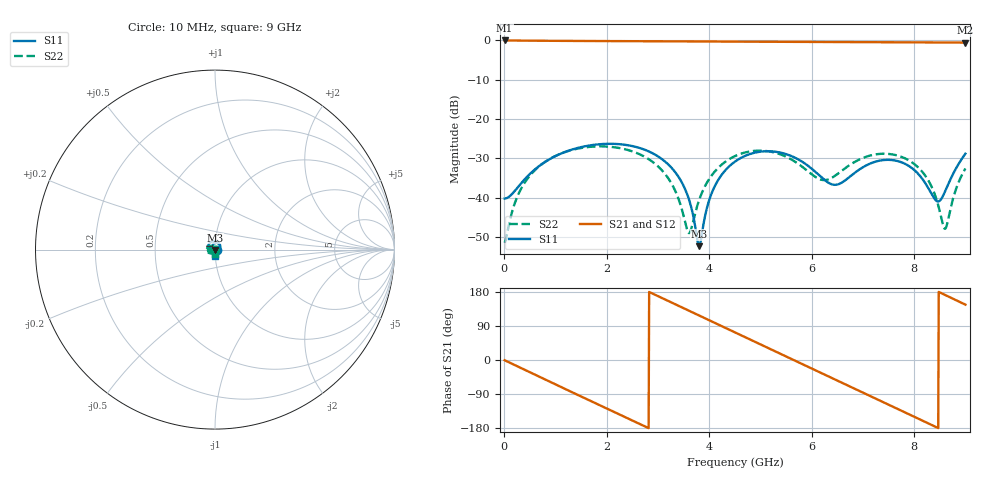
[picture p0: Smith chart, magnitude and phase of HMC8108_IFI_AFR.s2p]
! Analog Devices, Inc.
! 1 Analog Way
! Wilmington, MA 01887
! http://www.analog.com
! Date:  2021-09-07 NN
! Board Name:  EV1HMC8108LC5 Revision A with HMC8108LC5 installed
! File Description:  Automatic Fixture Removal S-Parameters for IFI Port connector and board loss de-embedding
! File Generation:  Calibrated Network Analyzer
! Chip Part Number:  HMC8108
! Chip Description:  X-Band, GaAs, MMIC, Low Noise Converter
! Chip Frequency:  9 to 10 GHz
! Chip Package:  LCC, 5 x 5 x 1.12 mm
! IFI Port:  HMC8108LC5 removed and end of trace left open
! Note:
!  Analog Devices supplies this data as a sample of measured data at the evaluation board
!  ports for this product.  Your particular data for this product may vary.
!  Analog Devices reserves the right to change this data at anytime.
!  All lines below in this file are as is from the Network Analyzer.
!Agilent Technologies,N5245A,MY52451809,A.10.47.06
!Automatic Fixture Removal (AFR)
!Date: Friday, August 27, 2021 5:28:33 AM
!S2P File: Measurements: S11,S21,S12,S22:
# MHz S  RI  R 50
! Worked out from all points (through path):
!   900 points, 10 MHz to 9 GHz, reference 50 ohm
!   highest |S21| = 0.00 dB at 10 MHz (marker M1); lowest = -0.5 dB at 9 GHz (marker M2)
!   group delay of S21, straight-line fit = 177 ps
!   lowest |S11| = -52.4 dB at 3.81 GHz (marker M3), VSWR 1.00, Z = 49.9 - j0.212 ohm
!   |S11| at or under -10 dB: start of sweep to end of sweep
!   |S22| runs from -51.5 to -27.0 dB; largest |S21 - S12| = 1.4e-15
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10  0.00969 -0.000508  1 -0.0112  1 -0.0112  -0.00264 -0.000366
230  0.00619 -0.011  0.964 -0.2547  0.964 -0.2547  -0.00429 -0.0082
500  -0.00511 -0.0192  0.8415 -0.5291  0.8415 -0.5291  -0.01 -0.016
1020  -0.0326 -0.0104  0.4099 -0.8993  0.4099 -0.8993  -0.0273 -0.0208
1510  -0.0389 0.0206  -0.1157 -0.9782  -0.1157 -0.9782  -0.0412 -0.0118
2330  0.0061 0.0468  -0.8377 -0.5078  -0.8377 -0.5078  -0.039 0.0145
3010  0.029 0.0163  -0.9544 0.201  -0.9544 0.201  -0.0156 0.0192
3330  0.0213 0.0015  -0.8233 0.5192  -0.8233 0.5192  -0.0063 0.0109
3600  0.00903 -0.00376  -0.6318 0.7382  -0.6318 0.7382  -0.00352 0.00045
3810  -0.00112 -0.00213  -0.443 0.8633  -0.443 0.8633  -0.00542 -0.00782
4080  -0.011 0.00636  -0.167 0.9539  -0.167 0.9539  -0.0126 -0.0159
4510  -0.0122 0.0261  0.2909 0.9207  0.2909 0.9207  -0.029 -0.0175
5300  0.0193 0.0331  0.8902 0.3615  0.8902 0.3615  -0.0366 0.00592
6010  0.0231 -0.000609  0.8807 -0.3743  0.8807 -0.3743  -0.0184 0.00671
6430  0.00437 -0.0139  0.6175 -0.7276  0.6175 -0.7276  -0.0181 -0.00355
6790  -0.0144 -0.0131  0.286 -0.9078  0.286 -0.9078  -0.0261 -0.00747
7510  -0.0293 0.00738  -0.4483 -0.8342  -0.4483 -0.8342  -0.0347 0.00936
8190  -0.0146 0.00714  -0.8959 -0.2962  -0.8959 -0.2962  -0.0101 0.0173
8440  -0.00875 -0.00219  -0.9419 -0.0367  -0.9419 -0.0367  -0.000201 0.0093
8600  -0.00586 -0.0103  -0.9325 0.1323  -0.9325 0.1323  0.0038 0.00124
8830  -0.00275 -0.0242  -0.8664 0.3663  -0.8664 0.3663  0.00464 -0.0127
9000  -0.000823 -0.0362  -0.7798 0.5242  -0.7798 0.5242  0.000858 -0.0234
